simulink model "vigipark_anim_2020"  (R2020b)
settings: Solver=ode45  StartTime=0.0  StopTime=inf  RelTol=1e-3  EnableMultiTasking=on
model workspace: external: MATLAB File (data not in the file)
undefined symbols (not defined in the file or in its folder): deg, kg, m, mm, N, s, smiData, X, Y, Z
libraries: sm_lib x10, nesl_utility x3, sldrtlib x1, simulink_extras x1

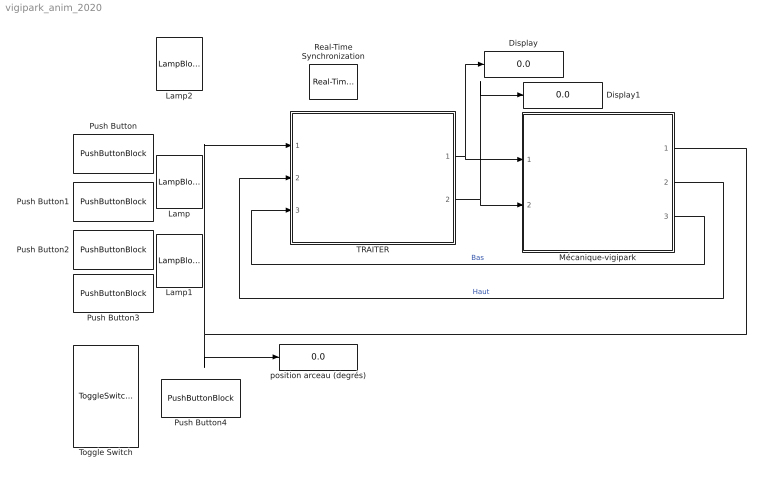
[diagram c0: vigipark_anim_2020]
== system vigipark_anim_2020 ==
  Display : Display
  Display1 : Display
  Lamp : LampBlock
  Lamp1 : LampBlock
  Lamp2 : LampBlock
  Mécanique-vigipark : Subsystem
  Push Button : PushButtonBlock  ButtonText=Marche
  Push Button1 : PushButtonBlock  ButtonText=Arrêt
  Push Button2 : PushButtonBlock  ButtonText=Descendre
  Push Button3 : PushButtonBlock  ButtonText=Monter
  Push Button4 : PushButtonBlock  ButtonText=Obstacle
  Real-Time Synchronization : sldrtlib/Real-Time Synchronization  SampleTime=0.1  MaxMissedTicks=10  ShowMissedTicks=off  YieldWhenWaiting=off
  TRAITER : Subsystem  mask{ON=0, OFF=0, Mont=0, Desc=0, Man_AUT=0, Obst=0}
      mask prompts: ON "BP_ON"; OFF "BP_OFF"; Mont "Monter"; Desc "Descendre"; Man_AUT "Manu/AUTO"; Obst "Obstacle"
  Toggle Switch : ToggleSwitchBlock  LabelPosition=Hide
  position arceau (degrés) : Display
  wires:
  Mécanique-vigipark/1(Pos_Arceau2) -> TRAITER/1(PosArceau), position arceau (degrés)/1
  TRAITER/2(Montee) -> Display1/1, Mécanique-vigipark/2(Monter)
  TRAITER/1(Descente) -> Display/1, Mécanique-vigipark/1(Descendre)
  Mécanique-vigipark/3(Bas1) -> TRAITER/3(Bas)  "Bas"
  Mécanique-vigipark/2(Haut1) -> TRAITER/2(Haut)  "Haut"

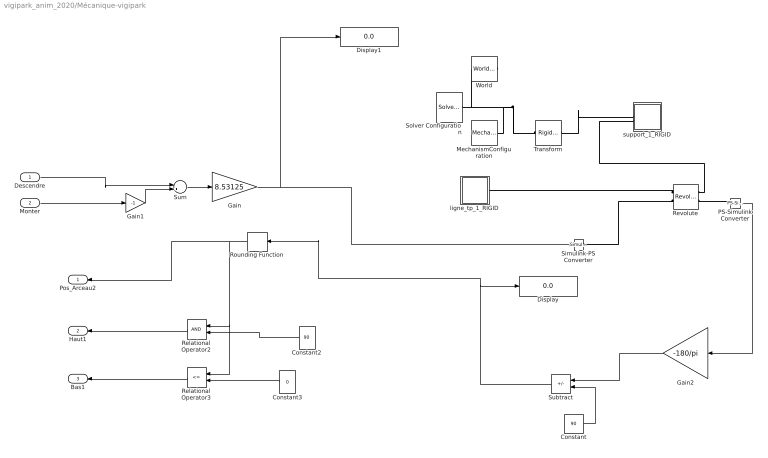
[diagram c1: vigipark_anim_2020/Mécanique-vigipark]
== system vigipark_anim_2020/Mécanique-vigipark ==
  Descendre : Inport
  Monter : Inport  Port=2
  Constant : Constant  Value=90
  Constant2 : Constant  Value=90
  Constant3 : Constant  Value=0
  Display : Display
  Display1 : Display
  Gain : Gain  Gain=8.53125
  Gain1 : Gain  Gain=-1
  Gain2 : Gain  Gain=-180/pi
  MechanismConfiguration : sm_lib/Utilities/Mechanism Configuration  UniformGravity=Constant  GravityVector=[0 -9.80665 0]  GravityVectorUnits=m/s^2  GravityUnits=m/s^2  LinearizationDelta=0.001  JointModeTransitionNonlinearIterations=2
  PS-Simulink Converter : nesl_utility/PS-Simulink Converter  PhysicalDomain=network_engine_domain  SubClassName=ps_output  LeftPortType=input  RightPortType=output  PseudoPeriodic=off  Frequencies=[]  Unit=inherit  AffineConversion=off
  Relational Operator2 : RelationalOperator  OutDataTypeStr=boolean
  Relational Operator3 : RelationalOperator  Operator=<=  OutDataTypeStr=boolean
  Revolute : sm_lib/Joints/Revolute Joint  JointMode=Normal  SenseConstraintForce=off  SenseConstraintForceX=off  SenseConstraintForceY=off  SenseConstraintForceZ=off  SenseConstraintTorque=off  SenseConstraintTorqueX=off  SenseConstraintTorqueY=off  SenseConstraintTorqueZ=off  SenseTotalForce=off  SenseTotalForceX=off  SenseTotalForceY=off  SenseTotalForceZ=off  SenseTotalTorque=off  SenseTotalTorqueX=off  SenseTotalTorqueY=off  SenseTotalTorqueZ=off  CompositeWrenchDir=FollowerOnBase  CompositeWrenchFrame=BaseFrame  EquilibriumPosition=0  EquilibriumPositionUnits=deg  SpringStiffness=0  SpringStiffnessUnits=N*m/deg  DampingCoefficient=2  DampingCoefficientUnits=N*m/(deg/s)  TorqueActuationMode=InputTorque  MotionActuationMode=ComputedMotion  SensePosition=on  SenseVelocity=off  SenseAcceleration=off  SenseTorqueForce=off  SenseLowerLimitTorqueForce=off  SenseUpperLimitTorqueForce=off  LowerLimitSpecify=off  LowerLimitBound=-90  LowerLimitBoundUnits=deg  LowerLimitStiffness=1e4  LowerLimitStiffnessUnits=N*m/deg  LowerLimitDamping=10  LowerLimitDampingUnits=N*m/(deg/s)  LowerLimitTransitionRegionWidth=0.1  LowerLimitTransitionRegionWidthUnits=deg  UpperLimitSpecify=off  UpperLimitBound=90  UpperLimitBoundUnits=deg  UpperLimitStiffness=1e4  UpperLimitStiffnessUnits=N*m/deg  UpperLimitDamping=10  UpperLimitDampingUnits=N*m/(deg/s)  UpperLimitTransitionRegionWidth=0.1  UpperLimitTransitionRegionWidthUnits=deg  PositionTargetSpecify=on  PositionTargetPriority=Low  PositionTargetValue=smiData.RevoluteJoint(1).Rz.Pos  PositionTargetValueUnits=deg  VelocityTargetSpecify=off  VelocityTargetPriority=High  VelocityTargetValue=0  VelocityTargetValueUnits=deg/s
  Rounding Function : Rounding  Operator=ceil
  Simulink-PS Converter : nesl_utility/Simulink-PS Converter  PhysicalDomain=network_engine_domain  SubClassName=ps_input  LeftPortType=input  RightPortType=output  PseudoPeriodic=off  Frequencies=[]  NoiseDistribution=none  NoiseParameters=[]  Unit=1  AffineConversion=off  FilteringAndDerivatives=provide  SimscapeFilterOrder=1  InputFilterTimeConstant=0.001  UdotUserProvided=0
  Solver Configuration : nesl_utility/Solver Configuration  PhysicalDomain=network_engine_domain  SubClassName=solver  LeftPortType=input  RightPortType=generic  Tones=[]  Harmonics=[]  SimulateNoise=off  Profile=off  UseLocalSampling=off  EnableSwitchedLinearOptims=on  FrequencyDomain=off  UseCCode=off  RelTol=0.001  AbsTol=1e-06  MinStep=1e-09  ToWorkspace=off  RevertToSquareIcSolve=off  NumHomotopyIterations=100  PhasorMode=off  PhasorModeNumHarmonics=1  DoDC=off  ResidualTolerance=1e-09  UseLocalSolver=off  LocalSolverChoice=NE_BACKWARD_EULER_ADVANCER  LocalSolverSampleTime=0.001  DoFixedCost=off  MaxNonlinIter=3  MaxModeIter=2  ComputeImpulses=off  ImpulseIterations=2  LinearAlgebra=auto  EquationFormulation=NE_TIME_EF  DelaysMemoryBudget=1024  AutomaticFiltering=on  FilteringTimeConstant=0.001  PartitionStorageMethod=AS_NEEDED  PartitionMemoryBudget=1024  PartitionMethod=ROBUST
  Subtract : Sum  Inputs=+-
  Sum : Sum  Inputs=|++
  Transform : sm_lib/Frames and Transforms/Rigid Transform  TranslationMethod=Cartesian  TranslationStandardOffset=0  TranslationLengthUnit=mm  TranslationStandardAxis=+Z  TranslationCartesianOffset=smiData.RigidTransform(3).translation  TranslationROffset=0  TranslationROffsetUnits=m  TranslationZOffset=0  TranslationZOffsetUnits=m  TranslationThetaOffset=0  TranslationThetaOffsetUnits=deg  RotationMethod=ArbitraryAxis  RotationAngleUnits=rad  RotationStandardAxis=+Z  RotationAngle=smiData.RigidTransform(3).angle  RotationArbitraryAxis=smiData.RigidTransform(3).axis  FollAlignAxisA=+X  BaseAlignAxisA=+Y  FollAlignAxisB=+Y  BaseAlignAxisB=+Z  RotationSequenceAxes=FollowerAxes  RotationSequence=XYX  RotationSequenceAngles=[0 0 0]  RotationSequenceAnglesUnits=deg  RotationMatrix=[1 0 0; 0 1 0; 0 0 1]
  World : sm_lib/Frames and Transforms/World Frame
  ligne_tp_1_RIGID : Subsystem
  support_1_RIGID : Subsystem
  Pos_Arceau2 : Outport
  Haut1 : Outport  Port=2
  Bas1 : Outport  Port=3
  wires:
  Sum/1 -> Gain/1
  Descendre/1 -> Sum/1
  Monter/1 -> Gain1/1
  Gain1/1 -> Sum/2
  Constant2/1 -> Relational Operator2/2
  PS-Simulink Converter/1 -> Gain2/1
  Relational Operator2/1 -> Haut1/1
  Relational Operator3/1 -> Bas1/1
  Constant3/1 -> Relational Operator3/2
  Gain/1 -> Display1/1, Simulink-PS Converter/1
  Gain2/1 -> Subtract/1
  Constant/1 -> Subtract/2
  Subtract/1 -> Display/1, Rounding Function/1
  Rounding Function/1 -> Relational Operator3/1, Relational Operator2/1, Pos_Arceau2/1
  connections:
  Solver Configuration/RConn1 -- World/RConn1 -- Transform/LConn1 -- MechanismConfiguration/RConn1
  Revolute/RConn1 -- support_1_RIGID/LConn2
  Simulink-PS Converter/RConn1 -- Revolute/LConn2
  PS-Simulink Converter/LConn1 -- Revolute/RConn2
  Revolute/LConn1 -- ligne_tp_1_RIGID/RConn1
  Transform/RConn1 -- support_1_RIGID/LConn1

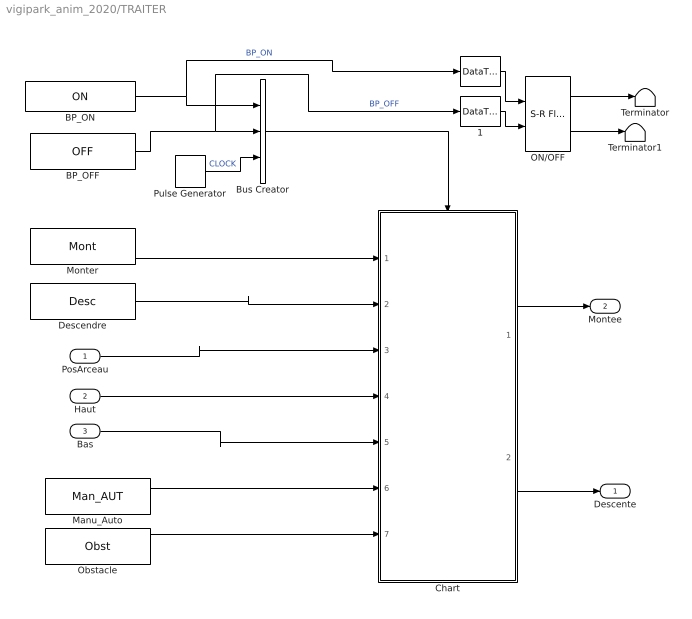
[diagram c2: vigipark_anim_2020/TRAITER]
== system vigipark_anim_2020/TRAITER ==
  PosArceau : Inport
  Haut : Inport  Port=2
  Bas : Inport  Port=3
  " " : DataTypeConversion  OutDataTypeStr=boolean
  1 : DataTypeConversion  OutDataTypeStr=boolean
  BP_OFF : Constant  Value=OFF
  BP_ON : Constant  Value=ON
  Bus Creator : BusCreator  Inputs=3
  Chart : Stateflow chart  TreatAsAtomicUnit=on
  Descendre : Constant  Value=Desc
  Manu_Auto : Constant  Value=Man_AUT
  Monter : Constant  Value=Mont
  ON/OFF : simulink_extras/Flip Flops/S-R Flip-Flop  initial_condition=0
  Obstacle : Constant  Value=Obst
  Pulse Generator : DiscretePulseGenerator  PulseType=Time based  Period=0.01  PulseWidth=50
  Terminator : Terminator
  Terminator1 : Terminator
  Descente : Outport
  Montee : Outport  Port=2
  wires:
  Descendre/1 -> Chart/2(Descendre)
  Monter/1 -> Chart/1(Monter)
  Chart/2(Baisser_arceau) -> Descente/1
  Chart/1(Lever_arceau) -> Montee/1
  Bus Creator/1 -> Chart/Trigger
  Pulse Generator/1 -> Bus Creator/3  "CLOCK"
  BP_OFF/1 -> 1/1, Bus Creator/2  "BP_OFF"
  BP_ON/1 -> " "/1, Bus Creator/1  "BP_ON"
  PosArceau/1 -> Chart/3(PosArceau)
  Manu_Auto/1 -> Chart/6(Manu_Auto)
  Obstacle/1 -> Chart/7(Obstacle)
  Bas/1 -> Chart/5(Bas)
  Haut/1 -> Chart/4(Haut)
  ON/OFF/1 -> Terminator/1
  ON/OFF/2 -> Terminator1/1
  " "/1 -> ON/OFF/1
  1/1 -> ON/OFF/2

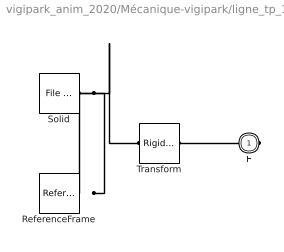
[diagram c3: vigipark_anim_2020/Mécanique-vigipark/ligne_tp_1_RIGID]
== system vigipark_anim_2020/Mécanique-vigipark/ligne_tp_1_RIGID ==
  ReferenceFrame : sm_lib/Frames and Transforms/Reference Frame
  Solid : sm_lib/Body Elements/File Solid  ExtGeomFileName=ligne_tp_Défaut_sldprt.STEP  UnitType=FromFile  ExtGeomFileUnits=m  StepReaderType=HEX  ExportConvexHullGeometry=off  InertiaType=Custom  Mass=smiData.Solid(1).mass  MassUnits=kg  CenterOfMass=smiData.Solid(1).CoM  CenterOfMassUnits=mm  MomentsOfInertia=smiData.Solid(1).MoI  MomentsOfInertiaUnits=kg*mm^2  ProductsOfInertia=smiData.Solid(1).PoI  ProductsOfInertiaUnits=kg*mm^2  BasedOnType=DensityFromFile  Density=1000  DensityUnits=kg/m^3  DoExposeReferenceFrame=on  SerializedFrames=<Frames/>  GraphicType=FromGeometry  MarkerShape=Sphere  MarkerSize=10  GraphicVisPropType=SimpleVisualProperties  GraphicDiffuseColor=smiData.Solid(1).color  GraphicSpecularColor=[0.5 0.5 0.5 1.0]  GraphicAmbientColor=[0.15 0.15 0.15 1.0]  GraphicEmissiveColor=[0.0 0.0 0.0 1.0]  GraphicShininess=75  GraphicOpacity=smiData.Solid(1).opacity
  Transform : sm_lib/Frames and Transforms/Rigid Transform  TranslationMethod=Cartesian  TranslationStandardOffset=0  TranslationLengthUnit=mm  TranslationStandardAxis=+Z  TranslationCartesianOffset=smiData.RigidTransform(1).translation  TranslationROffset=0  TranslationROffsetUnits=m  TranslationZOffset=0  TranslationZOffsetUnits=m  TranslationThetaOffset=0  TranslationThetaOffsetUnits=deg  RotationMethod=ArbitraryAxis  RotationAngleUnits=rad  RotationStandardAxis=+Z  RotationAngle=smiData.RigidTransform(1).angle  RotationArbitraryAxis=smiData.RigidTransform(1).axis  FollAlignAxisA=+X  BaseAlignAxisA=+Y  FollAlignAxisB=+Y  BaseAlignAxisB=+Z  RotationSequenceAxes=FollowerAxes  RotationSequence=XYX  RotationSequenceAngles=[0 0 0]  RotationSequenceAnglesUnits=deg  RotationMatrix=[1 0 0; 0 1 0; 0 0 1]
  F : PMIOPort  Side=Right
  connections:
  Solid/RConn1 -- ReferenceFrame/RConn1 -- Transform/LConn1
  Transform/RConn1 -- F/RConn1

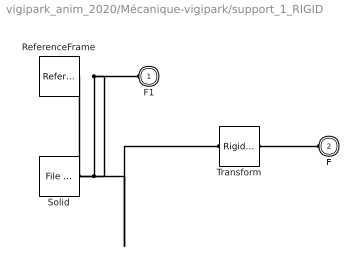
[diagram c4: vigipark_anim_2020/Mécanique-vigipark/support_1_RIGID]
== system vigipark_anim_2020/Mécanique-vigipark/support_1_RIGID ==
  ReferenceFrame : sm_lib/Frames and Transforms/Reference Frame
  Solid : sm_lib/Body Elements/File Solid  ExtGeomFileName=support_Défaut_sldprt.STEP  UnitType=FromFile  ExtGeomFileUnits=m  StepReaderType=HEX  ExportConvexHullGeometry=off  InertiaType=Custom  Mass=smiData.Solid(2).mass  MassUnits=kg  CenterOfMass=smiData.Solid(2).CoM  CenterOfMassUnits=mm  MomentsOfInertia=smiData.Solid(2).MoI  MomentsOfInertiaUnits=kg*mm^2  ProductsOfInertia=smiData.Solid(2).PoI  ProductsOfInertiaUnits=kg*mm^2  BasedOnType=DensityFromFile  Density=1000  DensityUnits=kg/m^3  DoExposeReferenceFrame=on  SerializedFrames=<Frames/>  GraphicType=FromGeometry  MarkerShape=Sphere  MarkerSize=10  GraphicVisPropType=SimpleVisualProperties  GraphicDiffuseColor=smiData.Solid(2).color  GraphicSpecularColor=[0.5 0.5 0.5 1.0]  GraphicAmbientColor=[0.15 0.15 0.15 1.0]  GraphicEmissiveColor=[0.0 0.0 0.0 1.0]  GraphicShininess=75  GraphicOpacity=smiData.Solid(2).opacity
  Transform : sm_lib/Frames and Transforms/Rigid Transform  TranslationMethod=Cartesian  TranslationStandardOffset=0  TranslationLengthUnit=mm  TranslationStandardAxis=+Z  TranslationCartesianOffset=smiData.RigidTransform(2).translation  TranslationROffset=0  TranslationROffsetUnits=m  TranslationZOffset=0  TranslationZOffsetUnits=m  TranslationThetaOffset=0  TranslationThetaOffsetUnits=deg  RotationMethod=ArbitraryAxis  RotationAngleUnits=rad  RotationStandardAxis=+Z  RotationAngle=smiData.RigidTransform(2).angle  RotationArbitraryAxis=smiData.RigidTransform(2).axis  FollAlignAxisA=+X  BaseAlignAxisA=+Y  FollAlignAxisB=+Y  BaseAlignAxisB=+Z  RotationSequenceAxes=FollowerAxes  RotationSequence=XYX  RotationSequenceAngles=[0 0 0]  RotationSequenceAnglesUnits=deg  RotationMatrix=[1 0 0; 0 1 0; 0 0 1]
  F1 : PMIOPort  Side=Left
  F : PMIOPort  Port=2  Side=Left
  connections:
  Solid/RConn1 -- ReferenceFrame/RConn1 -- Transform/LConn1 -- F1/RConn1
  Transform/RConn1 -- F/RConn1

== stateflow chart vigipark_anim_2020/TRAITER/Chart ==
  state VIGIPARK_ON
    state AUTOMATIQUE
    state Mode_Manuel
      state ARRETE
        entry:
        Baisser_arceau=0;
        Lever_arceau=0;
      (default) -> ARRETE
      ARRETE -> ARRETE : [(Descendre==1)&(Bas==0)]
    (default) -> AUTOMATIQUE : [Manu_Auto==1]
    (default) -> Mode_Manuel : [Manu_Auto==0]
  state VIGIPARK_OFF
  VIGIPARK_OFF -> VIGIPARK_ON : Marche
  VIGIPARK_ON -> VIGIPARK_OFF : Arret
  (default) -> VIGIPARK_OFF
  data: Monter input; Descendre input; Lever_arceau output double; Baisser_arceau output double; PosArceau input; Haut input; Bas input; Manu_Auto input; Obstacle input
  events: input RISING_EDGE_EVENT; input RISING_EDGE_EVENT; input RISING_EDGE_EVENT
